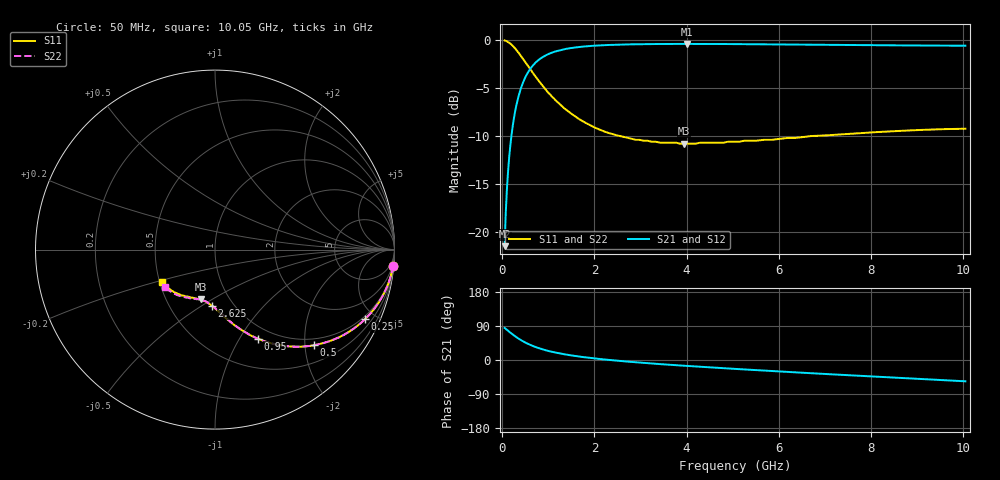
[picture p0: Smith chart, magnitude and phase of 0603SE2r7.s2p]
! AVX Thin Film Operation		Date: August 2001
! Description: Accu-P® Series, Thin Film, SMD, RF Capacitor
! Part Number: 06035J2R7ABT
! 50 MHz  -  10.05 GHz
! Serial Measurements
# mhz S db R 50
!	S11		S21		S12		S22
!	dB	Phase	dB	Phase	dB	Phase	dB	Phase
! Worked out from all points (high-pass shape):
!   401 points, 50 MHz to 10.05 GHz, reference 50 ohm
!   highest |S21| = -0.39 dB at 4 GHz (marker M1); lowest = -21.5 dB at 50 MHz (marker M2)
!   |S21| within 3 dB of the highest: 553 MHz to end of sweep
!   lowest |S11| = -10.8 dB at 3.95 GHz (marker M3), VSWR 1.81, Z = 36.9 - j22.3 ohm
!   |S11| at or under -10 dB: 2.55 GHz to 6.723 GHz (4.173 GHz wide, 90 % of centre)
!   |S22| runs from -10.7 to 0.0 dB; largest |S21 - S12| = 0
!   S11 on the Smith chart (normalised r, x): 50 MHz: 1, -22; 250 MHz: 0.85, -4.37; 500 MHz: 0.85, -2.20; 950 MHz: 0.84, -1.20; 2.625 GHz: 0.79, -0.55; 10.05 GHz: 0.52, -0.21
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50  -0.03 -5.3  -21.50 84.7  -21.50 84.7  -0.03 -5.3
75  -0.07 -7.9  -18.01 82.1  -18.01 82.1  -0.07 -7.9
125  -0.19 -13.0  -13.70 77.0  -13.70 77.0  -0.19 -13.0
150  -0.27 -15.5  -12.18 74.5  -12.18 74.5  -0.27 -15.5
200  -0.47 -20.3  -9.90 69.7  -9.90 69.7  -0.47 -20.3
250  -0.71 -24.9  -8.21 65.1  -8.21 65.1  -0.71 -24.9
350  -1.29 -33.4  -5.90 56.6  -5.90 56.6  -1.29 -33.4
500  -2.29 -43.9  -3.87 46.1  -3.87 46.1  -2.29 -43.9
600  -2.98 -49.7  -3.04 40.3  -3.04 40.3  -2.98 -49.7
725  -3.83 -55.8  -2.33 34.1  -2.33 34.1  -3.83 -55.8
950  -5.19 -64.4  -1.57 25.6  -1.57 25.6  -5.19 -64.4
1300  -6.92 -73.8  -0.99 16.1  -0.99 16.1  -6.92 -73.8
1725  -8.40 -81.8  -0.68 8.2  -0.68 8.2  -8.40 -81.6
2175  -9.46 -88.2  -0.53 1.9  -0.53 1.9  -9.45 -87.8
2625  -10.08 -93.3  -0.45 -3.2  -0.45 -3.2  -10.08 -92.8
3400  -10.68 -100.8  -0.40 -10.6  -0.40 -10.6  -10.68 -99.8
3950  -10.80 -106.0  -0.39 -15.2  -0.39 -15.2  -10.70 -104.1
4000  -10.80 -106.0  -0.39 -15.6  -0.39 -15.6  -10.70 -104.7
5050  -10.60 -114.0  -0.41 -23.5  -0.41 -23.5  -10.60 -112.0
6725  -10.00 -126.0  -0.47 -34.9  -0.47 -34.9  -10.00 -123.0
8400  -9.53 -138.1  -0.54 -45.9  -0.54 -45.9  -9.49 -133.1
10050  -9.24 -148.8  -0.58 -56.2  -0.58 -56.2  -9.20 -142.8
